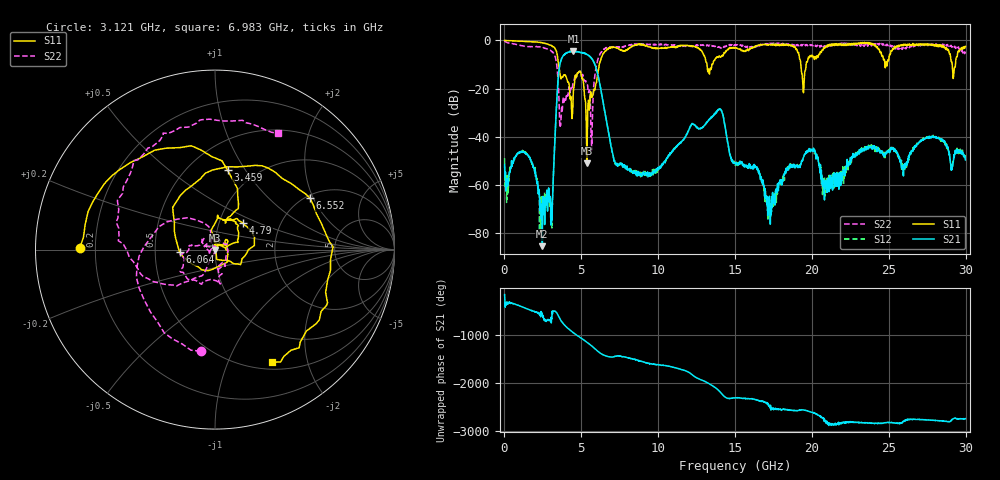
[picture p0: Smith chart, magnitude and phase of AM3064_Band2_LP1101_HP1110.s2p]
# Hz S DB R 50.0
!freq dBS11 angS11 dBS21 angS21 dBS12 angS12 dBS22 angS22
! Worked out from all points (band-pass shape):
!   1600 points, 10 MHz to 29.98 GHz, reference 50 ohm
!   highest |S21| = -4.41 dB at 4.49 GHz (marker M1); lowest = -85.3 dB at 2.465 GHz (marker M2)
!   |S21| within 3 dB of the highest: 3.73 GHz to 5.661 GHz (1.93 GHz wide, 41.1 % of centre)
!   lowest |S11| = -51.0 dB at 5.352 GHz (marker M3), VSWR 1.01, Z = 50 - j0.281 ohm
!   |S11| at or under -10 dB: 3.518 GHz to 6.165 GHz (2.647 GHz wide, 54.7 % of centre); 13.17 GHz to 13.49 GHz (320 MHz wide, 2.4 % of centre); 19.28 GHz to 19.62 GHz (344.3 MHz wide, 1.77 % of centre)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
!   |S22| runs from -45.5 to -0.2 dB; largest |S21 - S12| = 0.017
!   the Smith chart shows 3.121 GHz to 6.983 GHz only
!   S11 on the Smith chart (normalised r, x): 3.121 GHz: 0.14, +0.01; 3.459 GHz: 0.75, +0.83; 4.79 GHz: 1.30, +0.40; 6.064 GHz: 0.67, -0.02; 6.552 GHz: 2.11, +1.89; 6.983 GHz: 0.59, -1.46
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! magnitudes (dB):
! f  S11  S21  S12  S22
! 10 MHz  -0.1  -51.5  -48.9  -0.2
! 1.472 GHz  -0.5  -47.4  -47.0  -2.6
! 2.465 GHz  -1.0  -85.3  -69.8  -3.1
! 3.121 GHz  -2.5  -65.6  -68.1  -4.9
! 3.459 GHz  -7.0  -19.0  -18.9  -14.2
! 3.721 GHz  -15.3  -7.5  -7.5  -27.8
! 4.49 GHz  -20.6  -4.4  -4.6  -17.1
! 4.79 GHz  -13.3  -4.8  -4.7  -13.8
! 5.015 GHz  -14.9  -5.1  -5.1  -15.0
! 5.352 GHz  -51.0  -5.8  -5.8  -17.6
! 5.689 GHz  -23.6  -7.8  -7.7  -43.0
! 6.064 GHz  -14.1  -13.9  -13.9  -8.1
! 6.552 GHz  -4.4  -30.5  -30.5  -3.5
! 6.983 GHz  -3.1  -45.6  -45.4  -2.7
! 10 GHz  -3.4  -52.7  -53.9  -1.8
! 13.97 GHz  -6.6  -28.7  -28.5  -2.8
! 15 GHz  -2.9  -50.9  -51.0  -1.9
! 17.24 GHz  -1.7  -64.6  -69.5  -1.4
! 19.99 GHz  -6.1  -45.2  -45.5  -1.9
! 20.83 GHz  -3.2  -60.8  -64.7  -2.2
! 25 GHz  -8.0  -45.7  -45.4  -1.7
! 29.98 GHz  -2.5  -49.6  -49.8  -4.6
